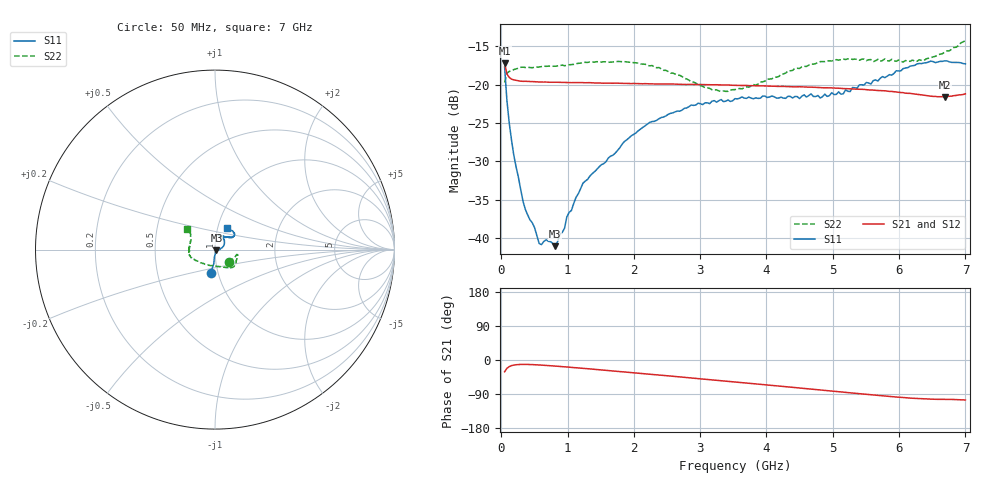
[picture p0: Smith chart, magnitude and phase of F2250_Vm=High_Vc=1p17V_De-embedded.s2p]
! Integrated Device Technology
! Corporate Headquarters
! 6024 Silver Creek Valley Road
! San Jose, CA 95138  USA
! Phone:  1-408-284-8200
! Toll Free:  1-800-223-1366
! Webpage:  http://www.idt.com/
! Timing and RF Division
! 515 Groton Road, Suite 102
! Westford, MA 01886-6024
! Device:  F2250
! Description: Voltage Variable RF Attenuator
! Frequency:  50.0 -  6000.00 MHz
! Package:  3x3 mm Thin QFN Plastic Package: 16 pin
! Ports:  2 RF, 3 DC
!  Pin  1  = GND
!  Pin  2  = NC
!  Pin  3  = RF1  = Port 1
!  Pin  4  = NC
!  Pin  5  = GND
!  Pin  6  = GND
!  Pin  7  = GND
!  Pin  8  = GND
!  Pin  9  = NC
!  Pin 10  = RF2  = Port 2
!  Pin 11  = NC
!  Pin 12  = GND
!  Pin 13  = GND
!  Pin 14  = VCNTRL
!  Pin 15  = VDD
!  Pin 16  = VMODE
! Vcntrl:  1.170 Volts
! Vmode:  +3.300 Volts
! Vdd:  +3.30  Volts
! Current:  1.331 mA
! Data:  The device was measured on a the F2250 evaluation board which has
!  individual transmission lines to the RF pins.  Data was collected
!  using a calibrated network analyzer.  The evaluation board was
!  de-embedded using a TRL calibration technique.
!  The reference plane is the edge of the package pin.
! Misc:  SN 10
!  Action Tracker AT0258
! Date Measured:  2014-11-26
! Date:  2015-10-15  MJV
! Note:
!  Integrated Device Technology supplies this data as a sample of measured
!  data at the package pin for this product.  Your particular data for this
!  product may vary.
!  Data was taken at 25 degrees C.
!  Integrated Device Technology reserves the right to change this data at anytime.
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# GHz S dB R 50
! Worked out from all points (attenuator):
!   201 points, 50 MHz to 7 GHz, reference 50 ohm
!   highest |S21| = -17.23 dB at 50 MHz (marker M1); lowest = -21.6 dB at 6.687 GHz (marker M2)
!   lowest |S11| = -41.0 dB at 814.5 MHz (marker M3), VSWR 1.02, Z = 50.8 - j0.324 ohm
!   |S11| at or under -10 dB: start of sweep to end of sweep
!   |S22| runs from -20.9 to -14.2 dB; largest |S21 - S12| = 0.00043
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0.05  -17.70 -100.5  -17.23 -31.1  -17.24 -31.1  -19.71 -42.8
0.08475  -22.05 -94.9  -18.59 -22.1  -18.57 -22.0  -18.51 -21.2
0.15425  -27.23 -94.9  -19.27 -14.9  -19.25 -14.8  -18.18 -13.1
0.328  -35.21 -81.5  -19.56 -11.6  -19.54 -11.6  -17.71 -12.7
0.50175  -38.63 -64.6  -19.61 -12.4  -19.59 -12.4  -17.73 -16.2
0.57125  -40.70 -51.0  -19.65 -13.1  -19.63 -13.1  -17.70 -17.8
0.6755  -40.21 -44.9  -19.65 -14.3  -19.66 -14.3  -17.60 -20.0
0.8145  -41.05 -21.1  -19.69 -16.1  -19.68 -16.1  -17.59 -23.8
0.9535  -38.72 -23.8  -19.70 -17.9  -19.71 -17.9  -17.53 -27.4
0.98825  -37.25 -20.6  -19.71 -18.4  -19.73 -18.4  -17.48 -28.1
1.05775  -36.39 -14.3  -19.73 -19.4  -19.71 -19.4  -17.38 -28.9
1.2315  -32.84 -3.1  -19.73 -21.9  -19.72 -22.0  -17.09 -33.2
1.857  -27.40 16.6  -19.83 -31.5  -19.81 -31.5  -16.99 -43.1
2.37825  -24.44 30.3  -19.91 -39.6  -19.91 -39.6  -17.76 -52.1
3.1775  -22.15 52.9  -20.01 -52.4  -20.02 -52.5  -20.66 -84.7
3.525  -21.81 63.5  -20.07 -58.1  -20.07 -58.1  -20.64 -108.8
4.7065  -21.53 68.0  -20.34 -77.4  -20.34 -77.4  -17.32 -159.3
5.15825  -21.19 51.4  -20.50 -84.8  -20.48 -84.9  -16.66 -168.4
5.85325  -18.68 36.5  -20.87 -96.0  -20.85 -96.2  -16.90 176.0
6.3745  -17.16 38.2  -21.37 -102.7  -21.36 -102.8  -16.85 158.3
6.68725  -16.90 45.8  -21.59 -103.9  -21.57 -104.1  -15.77 146.8
7  -17.28 62.0  -21.19 -105.5  -21.18 -105.7  -14.23 143.6
